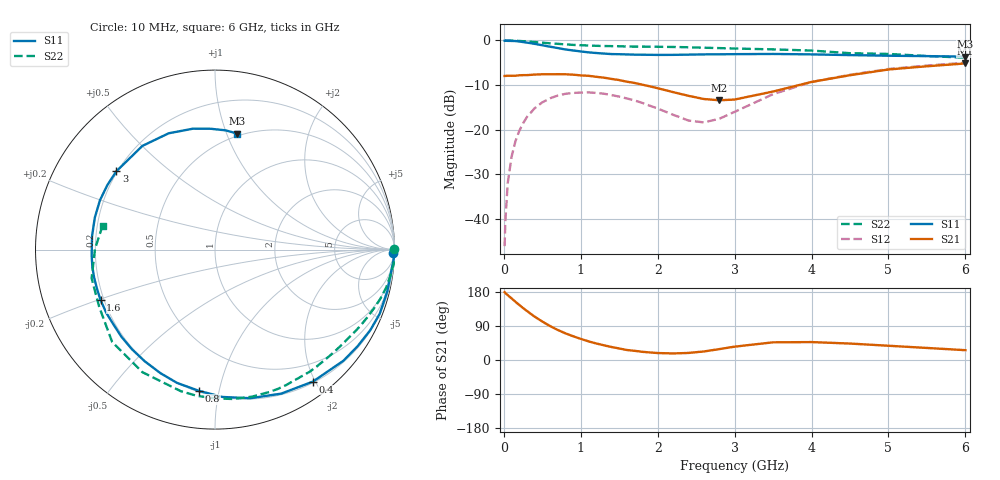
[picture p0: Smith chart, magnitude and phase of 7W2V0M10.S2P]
! Infineon Technologies  Discrete & RF Semiconductors
! BFS17W
! Si NPN RF Bipolar Junction Transistor in SOT323
! VCE = 2 V  IC = 0.1 mA
! Common Emitter S-Parameters:  August  1999
# GHz  S  MA  R  50
!  f  S11  S21  S12  S22
! GHz  MAG  ANG  MAG  ANG  MAG  ANG  MAG  ANG
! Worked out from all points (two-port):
!   36 points, 10 MHz to 6 GHz, reference 50 ohm
!   highest |S21| = -5.16 dB at 6 GHz (marker M1); lowest = -13.4 dB at 2.8 GHz (marker M2)
!   |S21| within 3 dB of the highest: start of sweep to 1.202 GHz; 4.383 GHz to end of sweep
!   lowest |S11| = -3.6 dB at 6 GHz (marker M3), VSWR 4.85, Z = 23.8 + j54.4 ohm
!   |S11| at or under -10 dB: nowhere
!   |S22| runs from -3.9 to 0.0 dB; largest |S21 - S12| = 0.4
!   S11 on the Smith chart (normalised r, x): 10 MHz: 29, -86; 400 MHz: 0.22, -1.97; 800 MHz: 0.21, -0.87; 1.6 GHz: 0.19, -0.20; 3 GHz: 0.20, +0.34; 6 GHz: 0.48, +1.09
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0.01  0.993 -1.2  0.399 179.1  0.0049 87.1  0.9999 0.1
0.02  0.9972 -2.9  0.399 176.6  0.0094 89.9  0.9926 -0.8
0.05  0.9892 -6.9  0.402 171.3  0.0248 85.9  0.9985 -2.2
0.1  0.9876 -13.6  0.401 162.7  0.0493 81.3  0.999 -4.5
0.2  0.9746 -27.5  0.406 145.4  0.0963 72.0  0.9875 -8.7
0.3  0.9464 -40.8  0.408 129.4  0.1381 63.2  0.9758 -12.8
0.4  0.9158 -53.4  0.414 114.4  0.1732 54.9  0.9601 -16.8
0.6  0.8511 -76.6  0.417 89.6  0.2239 40.9  0.9293 -23.8
0.8  0.7919 -96.5  0.417 70.4  0.2515 29.5  0.9038 -30.4
1.1  0.7351 -122.2  0.401 49.2  0.2612 15.9  0.8771 -39.6
1.3  0.7126 -137.0  0.382 38.8  0.2524 8.9  0.8657 -46.1
1.6  0.6969 -156.1  0.344 26.4  0.2232 1.5  0.8552 -55.6
2.2  0.6891 173.8  0.263 17.3  0.1465 4.5  0.8448 -76.0
2.6  0.6975 156.7  0.22 22.5  0.1202 29.2  0.8286 -90.1
2.8  0.6992 148.9  0.213 28.7  0.1319 43.7  0.8208 -97.1
3  0.7017 141.5  0.217 35.2  0.1579 53.8  0.8116 -103.5
3.5  0.7053 125.0  0.267 46.6  0.2495 60.6  0.7938 -120.6
4  0.6975 111.7  0.342 47.3  0.3419 55.6  0.7701 -138.1
4.5  0.6848 100.4  0.407 43.4  0.4121 48.2  0.7193 -153.9
5  0.6736 92.0  0.472 37.6  0.4781 41.0  0.7057 -166.9
5.5  0.667 84.9  0.513 31.8  0.5226 34.1  0.6689 179.7
6  0.6582 79.3  0.552 25.9  0.5624 27.8  0.6403 168.0
